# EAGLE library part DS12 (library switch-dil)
DIL/CODE SWITCH
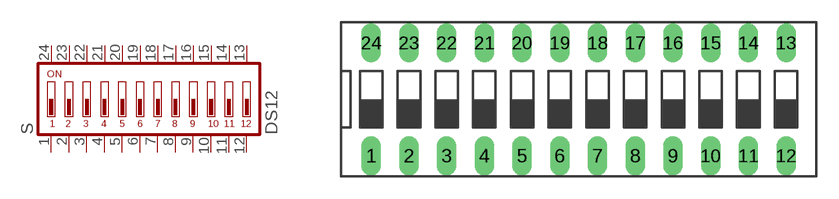
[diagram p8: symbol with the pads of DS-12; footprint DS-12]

Designator prefix S

## DS12 (OC_FARNELL: unknown; OC_NEWARK: unknown)  [DS-12]
1  1  pas
2  2  pas
3  3  pas
4  4  pas
5  5  pas
6  6  pas
7  7  pas
8  8  pas
9  9  pas
10  10  pas
11  11  pas
12  12  pas
13  13  pas
14  14  pas
15  15  pas
16  16  pas
17  17  pas
18  18  pas
19  19  pas
20  20  pas
21  21  pas
22  22  pas
23  23  pas
24  24  pas

## Footprint DS-12 (pad centres in mm)
DIL/CODE SWITCH Mors distributor Buerklin, 17G568
drill 0.813 long: 1 -13.97,-3.81; 2 -11.43,-3.81; 3 -8.89,-3.81; 4 -6.35,-3.81; 5 -3.81,-3.81; 6 -1.27,-3.81; 7 1.27,-3.81; 8 3.81,-3.81; 9 6.35,-3.81; 10 8.89,-3.81; 11 11.43,-3.81; 12 13.97,-3.81; 13 13.97,3.81; 14 11.43,3.81; 15 8.89,3.81; 16 6.35,3.81; 17 3.81,3.81; 18 1.27,3.81; 19 -1.27,3.81; 20 -3.81,3.81; 21 -6.35,3.81; 22 -8.89,3.81; 23 -11.43,3.81; 24 -13.97,3.81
